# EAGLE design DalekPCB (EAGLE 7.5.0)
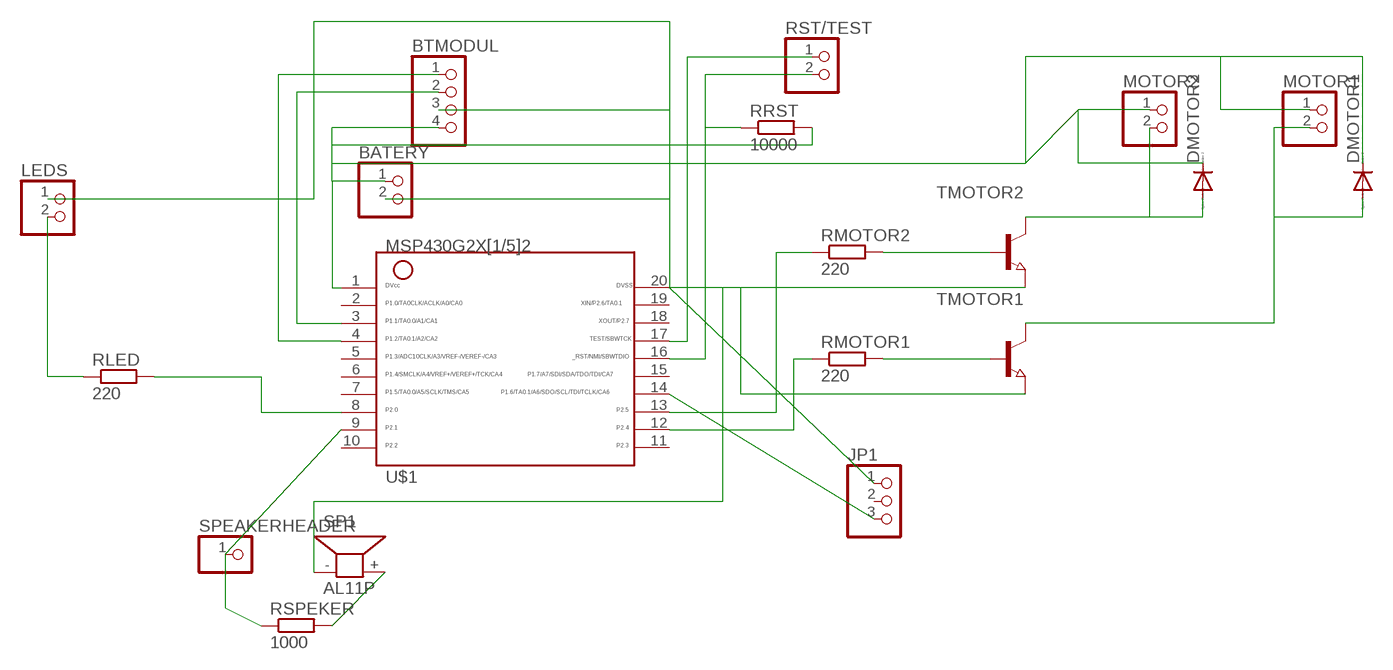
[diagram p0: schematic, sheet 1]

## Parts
BATERY  PINHD-1X2  [1X02]
BTMODUL  PINHD-1X4/90  [1X04/90]
DMOTOR1  DIODE-SOD323-W  [SOD323-W]
DMOTOR2  DIODE-SOD323-W  [SOD323-W]
JP1  PINHD-1X3  [1X03]
LEDS  PINHD-1X2  [1X02]
MOTOR1  PINHD-1X2  [1X02]
MOTOR2  PINHD-1X2  [1X02]
RLED  220  R-EU_R1206  [R1206]
RMOTOR1  220  R-EU_R1206  [R1206]
RMOTOR2  220  R-EU_R1206  [R1206]
RRST  10000  R-EU_0204/2V  [0204V]
RSPEKER  1000  R-EU_0204/2V  [0204V]
RST/TEST  PINHD-1X2  [1X02]
SP1  AL11P  [AL11P]
SPEAKERHEADER  PINHD-1X1  [1X01]
TMOTOR1  NPN-TRANSISTOR_SOT23  [SOT23]
TMOTOR2  NPN-TRANSISTOR_SOT23  [SOT23]
U$1  G2X[1/5]2---N20  [N20]

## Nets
N$1: RSPEKER.1 SPEAKERHEADER.1 U$1.9
N$2: BATERY.2 BTMODUL.3 JP1.1 LEDS.1 SP1.- TMOTOR1.2(E) TMOTOR2.2(E) U$1.20
N$3: RLED.2 U$1.8
N$4: LEDS.2 RLED.1
N$5: BATERY.1 BTMODUL.4 DMOTOR1.C DMOTOR2.C MOTOR1.1 MOTOR2.1 RRST.2 U$1.1
N$6: BTMODUL.2 U$1.3
N$7: BTMODUL.1 U$1.4
N$8: RMOTOR2.1 U$1.13
N$9: RMOTOR1.1 U$1.12
N$10: RMOTOR2.2 TMOTOR2.1(B)
N$11: RMOTOR1.2 TMOTOR1.1(B)
N$12: DMOTOR2.A MOTOR2.2 TMOTOR2.3(C)
N$13: JP1.3 U$1.14
N$14: DMOTOR1.A MOTOR1.2 TMOTOR1.3(C)
N$18: RSPEKER.2 SP1.+
N$20: RST/TEST.1 U$1.17
N$21: RRST.1 RST/TEST.2 U$1.16
Unconnected: JP1.2 U$1.2 U$1.5 U$1.6 U$1.7 U$1.10 U$1.11 U$1.15 U$1.18 U$1.19

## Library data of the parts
BATERY LEDS MOTOR1 MOTOR2 RST/TEST = pinhead:PINHD-1X2: PIN HEADER
BTMODUL = pinhead:PINHD-1X4: PIN HEADER
DMOTOR1 DMOTOR2 = diode:DIODE-: DIODE
JP1 = pinhead:PINHD-1X3: PIN HEADER
RLED RMOTOR1 RMOTOR2 = rcl:R-EU_: RESISTOR, European symbol
RRST RSPEKER = resistor:R-EU_: RESISTOR, European symbol
SP1 = buzzer:AL11P: SPEAKER; OC_FARNELL: unknown; OC_NEWARK: unknown
SPEAKERHEADER = pinhead:PINHD-1X1: PIN HEADER
TMOTOR1 TMOTOR2 = semicon-smd-ipc:NPN-TRANSISTOR_: NPN TRANSISTOR
U$1 = TI_MSP430_v16:G2X[1/5]2---N20: MSP430G2X[1/5]2 MSP430G2x52, MSP430G2x12 PDIP (N) 20 Pin Package http://focus.ti.com/docs/prod/folders/print/msp430g2452.html

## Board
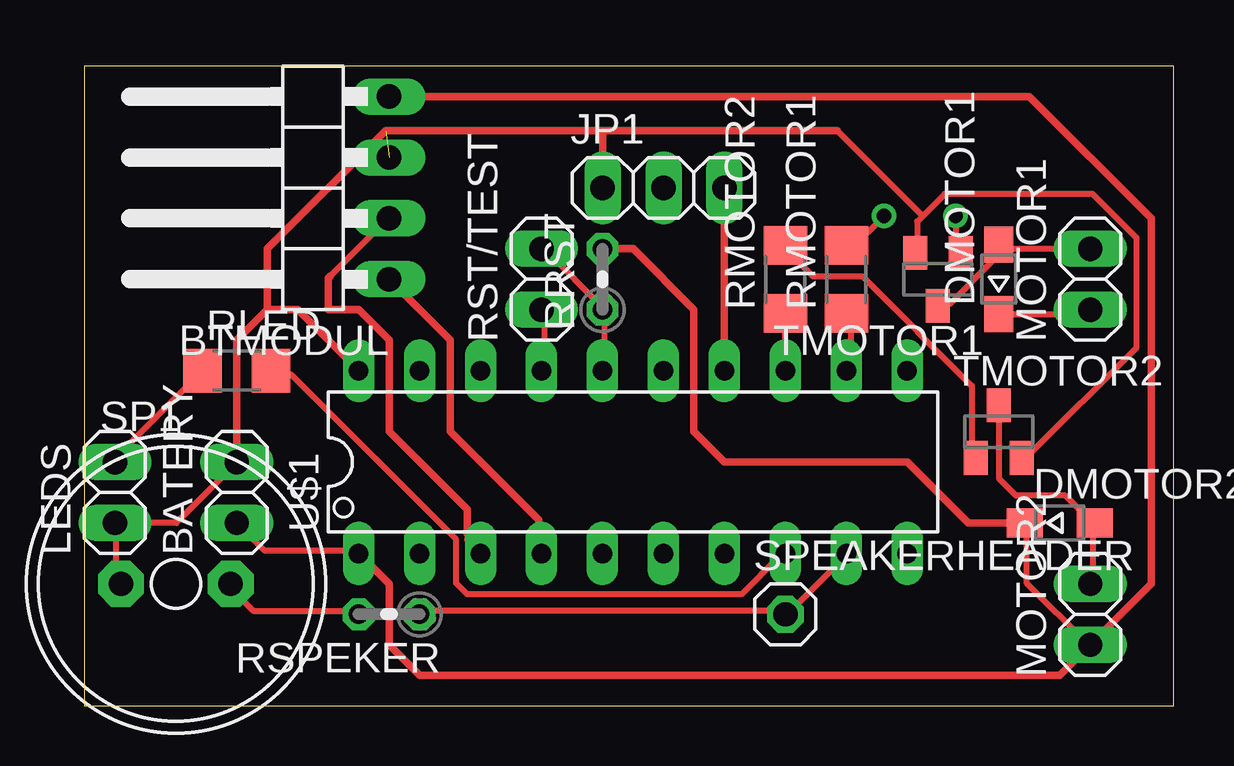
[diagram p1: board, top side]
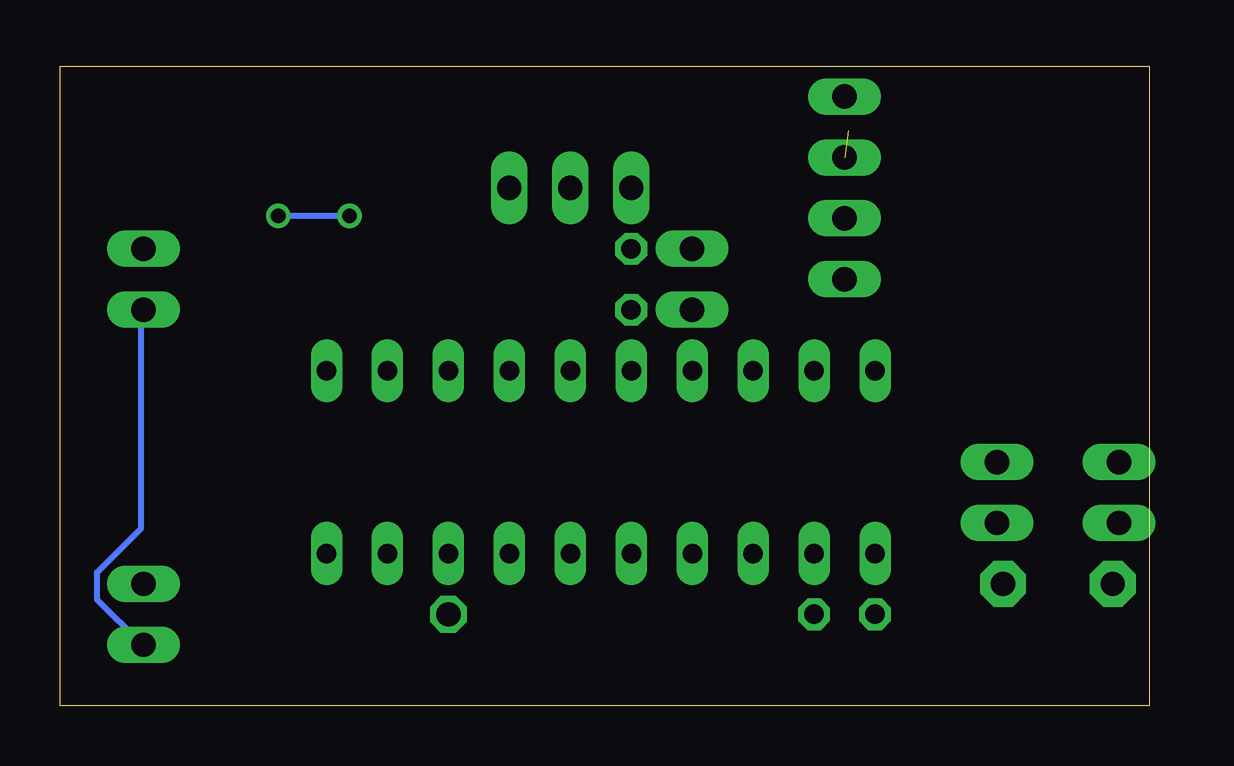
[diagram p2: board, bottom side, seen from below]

Size 45.39 x 26.66 mm. Coordinates in mm from the lower left corner, seen from the top.
Outline: 0,0 45.39,0 45.39,26.66 0,26.66 0,0
Copper layers (1*16): Top 0.035mm / dielectric 1.5mm / Bottom 0.035mm
Design rules "default": minimum track width 10mil, minimum drill 24mil, track to track 8mil, track to pad 8mil, pad to pad 8mil, via to via 8mil, smd to smd 8mil, copper to edge 40mil, drill to drill 8mil, minimum pad ring 10mil, minimum via ring 8mil, stop-mask expansion 4mil, vias tented up to drill 0mil, thermal gap 10mil

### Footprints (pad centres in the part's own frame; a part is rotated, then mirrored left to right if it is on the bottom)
1X02 = drill 1.016 long: 1 -1.27,0; 2 1.27,0
1X04/90 = drill 1.016 long: 1 -3.81,-3.81; 2 -1.27,-3.81; 3 1.27,-3.81; 4 3.81,-3.81
SOD323-W = smd 1.5 x 1.2: A 1.45,0; C -1.45,0
1X03 = drill 1.016 long: 1 -2.54,0; 2 0,0; 3 2.54,0
R1206 = smd 1.6 x 1.803: 1 -1.422,0; 2 1.422,0
0204V = drill 0.813 octagon: 1 -1.27,0; 2 1.27,0
AL11P = drill 1.016 pad 1.905 octagon: + 2.286,0; - -2.286,0
1X01 = drill 1.016 octagon: 1 0,0
SOT23 = smd 1 x 1.4: 1 -0.95,-1.1; 2 0.95,-1.1; 3 0,1.1
N20 = drill 0.813 long: 1 -11.435,-3.81; 2 -8.895,-3.81; 3 -6.355,-3.81; 4 -3.815,-3.81; 5 -1.275,-3.81; 6 1.265,-3.81; 7 3.805,-3.81; 8 6.345,-3.81; 9 8.885,-3.81; 10 11.425,-3.81; 11 11.425,3.81; 12 8.885,3.81; 13 6.345,3.81; 14 3.805,3.81; 15 1.265,3.81; 16 -1.275,3.81; 17 -3.815,3.81; 18 -6.355,3.81; 19 -8.895,3.81; 20 -11.435,3.81

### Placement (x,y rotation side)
BATERY  6.35,8.89 90 top
BTMODUL  8.89,21.59 90 top
DMOTOR1  38.1,17.78 90 top
DMOTOR2  40.64,7.62 0 top
JP1  24.13,21.59 0 top
LEDS  1.27,8.89 90 top
MOTOR1  41.91,17.78 90 top
MOTOR2  41.91,3.81 90 top
RLED  6.35,13.97 0 top
RMOTOR1  31.75,17.78 90 top
RMOTOR2  29.21,17.78 90 top
RRST  21.59,17.78 90 top
RSPEKER  12.7,3.81 180 top
RST/TEST  19.05,17.78 90 top
SP1  3.81,5.08 0 top
SPEAKERHEADER  29.21,3.81 0 top
TMOTOR1  35.56,17.78 180 top
TMOTOR2  38.1,11.43 0 top
U$1  22.86,10.16 0 top

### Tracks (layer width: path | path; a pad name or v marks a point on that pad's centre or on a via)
N$1
  Top 0.254: RSPEKER.1 14.12,3.96 29.21,3.96 SPEAKERHEADER.1 29.21,3.73 31.72,6.25 U$1.9
N$2  (1 unrouted)
  Top 0.254: 34.92,20.42 35.84,21.34 42.01,21.34 43.84,19.51 43.84,14.93 39.27,10.36 TMOTOR2.2 | 34.92,20.42 34.7,20.19 34.7,19.05 TMOTOR1.2 | 1.32,7.62 1.32,5.1 SP1.- | 1.32,7.62 3.83,7.62 6.35,10.13 BATERY.2 | 1.32,7.62 LEDS.1 | 31.37,23.98 34.92,20.42
  Top 0.305: BATERY.2 6.35,15.24 7.62,16.51 | 7.62,16.51 8.89,16.51 U$1.20 | 7.62,16.51 7.62,19.05 12.55,23.98 21.59,23.98 | 31.37,23.98 21.59,23.98 | BTMODUL.3 11.43,22.86 11.28,22.71 | JP1.1 21.59,23.98
N$3
  Top 0.254: RLED.2 7.95,13.79 8.64,13.79 15.49,6.93 15.49,5.1 15.95,4.65 27.38,4.65 28.98,6.25 U$1.8
N$4
  Top 0.254: RLED.1 4.75,13.79 1.32,10.36 LEDS.2
N$5
  Top 0.254: DMOTOR1.C 38.12,16.31 41.78,16.31 MOTOR1.1 | DMOTOR2.C 39.27,7.62 39.27,5.1 41.78,2.59 MOTOR2.1 | BATERY.1 7.49,6.48 11.38,6.48 U$1.1
  Top 0.305: BTMODUL.4 39.37,25.4 44.45,20.32 44.45,5.08 MOTOR2.1 40.64,1.27 13.97,1.27 12.7,2.54 12.7,5.08 U$1.1 | RRST.2 22.86,19.05 25.4,16.51 25.4,11.43 26.67,10.16 34.29,10.16 36.83,7.62 DMOTOR2.C
  Bottom 0.254: MOTOR2.1 42.01,2.59 43.84,4.42 43.84,5.56 42.01,7.39 42.01,16.31 MOTOR1.1 41.78,16.53
N$6
  Top 0.254: 15.95,7.16 15.95,6.93 16.41,6.48 U$1.3 | 10.24,17.91 12.52,20.19 BTMODUL.2
  Top 0.305: 15.95,7.16 15.95,8.18 12.7,11.43 12.7,15.24 11.43,16.51 10.16,16.51 10.16,17.83 10.24,17.91
N$7
  Top 0.254: 18.92,6.93 18.92,6.48 U$1.4 | 12.75,17.68 BTMODUL.1
  Top 0.305: 18.92,6.93 18.92,7.75 15.24,11.43 15.24,15.24 BTMODUL.1
N$8
  Top 0.254: RMOTOR2.1 29.21,14.02 U$1.13
N$9
  Top 0.254: RMOTOR1.1 31.95,16.31 31.95,14.02 U$1.12
N$10
  Top 0.254: TMOTOR2.1 36.98,10.36 36.98,13.34 32.41,17.91 30.35,17.91 29.21,19.05 RMOTOR2.2
N$11  (via drill 0.61)
  Top 0.254: v36.3,20.42 36.3,19.05 TMOTOR1.1 | v33.33,20.42 31.95,19.05 RMOTOR1.2
  Bottom 0.254: v33.33,20.42 v36.3,20.42
N$12
  Top 0.254: 42.01,7.62 40.87,8.76 38.81,8.76 38.12,9.45 38.12,12.42 TMOTOR2.3 | 42.01,7.62 42.01,5.1 MOTOR2.2 | 42.01,7.62 DMOTOR2.A
N$13
  Top 0.305: U$1.14 JP1.3
N$14
  Top 0.254: TMOTOR1.3 35.61,16.76 36.07,16.76 37.9,18.59 37.9,19.05 DMOTOR1.A 38.12,19.05 MOTOR1.2
N$18
  Top 0.254: RSPEKER.2 11.38,3.96 7.04,3.96 6.12,4.88 SP1.+
N$20
  Top 0.254: U$1.17 19.15,14.02 19.15,16.31 RST/TEST.1
N$21
  Top 0.254: U$1.16 21.67,14.02 21.67,16.31 RRST.1 21.67,16.53 19.15,19.05 RST/TEST.2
